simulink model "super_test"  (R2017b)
settings: Solver=FixedStepDiscrete  StartTime=0.0  StopTime=10.0  FixedStep=0.01  RelTol=1e-3
undefined symbols (not defined in the file or in its folder): BCCR_tiPwrUpCondLv_C, bin2dec, HVSR_dcHvilPwmDutyHi_C, HVSR_dcHvilPwmDutyLo_C, HVSR_dcHvilPwmDutyNrm_C, HVSR_dcHvilPwmDutyOpl_C, HVSR_dcHvilPwmDutyOptSet_C, HVSR_dcHvilPwmDutyThres_C, HVSR_fHvilPwmFrqHi_C, HVSR_fHvilPwmFrqLo_C, HVSR_tiHvilOplErr_C, HVSR_tiHvilScbErr_C, HVSR_tiHvilScgErr_C, HVSR_uKL30ThresHi_C, HVSR_uKL30ThresLo_C
libraries: simulink x41

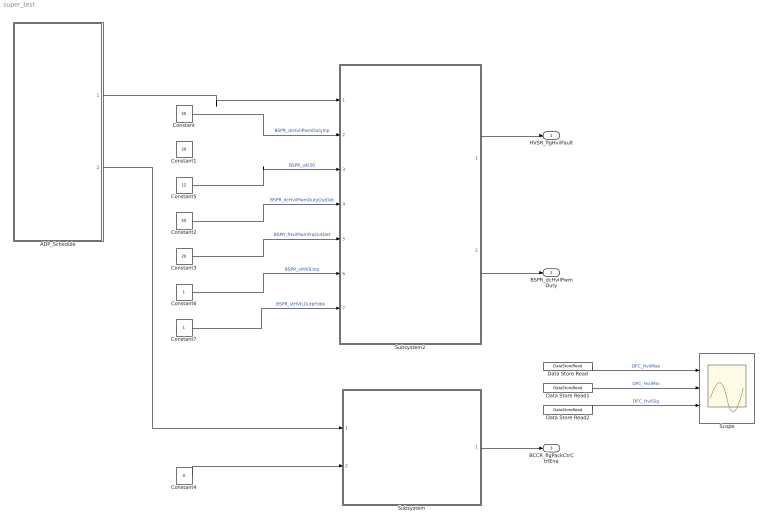
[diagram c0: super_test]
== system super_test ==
  ADP_Schedule : Stateflow chart  TreatAsAtomicUnit=on
  Constant : Constant  Value=50  OutDataTypeStr=single
  Constant1 : Constant  Value=20  OutDataTypeStr=single
  Constant2 : Constant  Value=50  OutDataTypeStr=single
  Constant3 : Constant  Value=20  OutDataTypeStr=single
  Constant4 : Constant  Value=0  OutDataTypeStr=boolean
  Constant5 : Constant  Value=12  OutDataTypeStr=single
  Constant6 : Constant  OutDataTypeStr=uint8
  Constant7 : Constant  OutDataTypeStr=uint8
  Data Store Read : DataStoreRead  DataStoreName=DFC_HvilMax
  Data Store Read1 : DataStoreRead  DataStoreName=DFC_HvilMin
  Data Store Read2 : DataStoreRead  DataStoreName=DFC_HvilSig
  Scope : Scope  NumInputPorts=3
  Subsystem : Subsystem
  Subsystem2 : Subsystem
  HVSR_flgHvilFault : Outport
  BSPR_dcHvilPwmDuty : Outport  Port=2
  BCCR_flgPackCtrCtrlEna : Outport  Port=3
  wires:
  Constant/1 -> Subsystem2/2(BSPR_dcHvilPwmDutyInp)  "BSPR_dcHvilPwmDutyInp"
  Constant1/1 -> ?  "BSPR_fHvilPwmFrq"
  Constant5/1 -> Subsystem2/3(BSPR_uKl30)  "BSPR_uKl30"
  Constant2/1 -> Subsystem2/4(BSPR_dcHvilPwmDutyOutDet)  "BSPR_dcHvilPwmDutyOutDet"
  Constant3/1 -> Subsystem2/5(BSPR_fHvilPwmFrqOutDet)  "BSPR_fHvilPwmFrqOutDet"
  Constant6/1 -> Subsystem2/6(BSPR_stHVILInp)  "BSPR_stHVILInp"
  Constant7/1 -> Subsystem2/7(BSPR_stHVILOutpFdbk)  "BSPR_stHVILOutpFdbk"
  Subsystem2/1(HVSR_flgHvilFault) -> HVSR_flgHvilFault/1
  Subsystem2/2(BSPR_dcHvilPwmDuty) -> BSPR_dcHvilPwmDuty/1
  Constant4/1 -> Subsystem/2(COMR_bKl30cLowDet)
  Subsystem/1(BCCR_flgPackCtrCtrlEna) -> BCCR_flgPackCtrCtrlEna/1
  ADP_Schedule/1(HVSR_HvilChk_step_10ms()) -> Subsystem2/1(HVSR_HvilChk_step)
  ADP_Schedule/2(BCCR_RlyCtlDiag_step_10ms()) -> Subsystem/1(BCCR_RlyCtlDiag_step)
  Data Store Read/1 -> Scope/1  "DFC_HvilMax"
  Data Store Read1/1 -> Scope/2  "DFC_HvilMin"
  Data Store Read2/1 -> Scope/3  "DFC_HvilSig"

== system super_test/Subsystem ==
  BCCR_RlyCtlDiag_step : Inport
  COMR_bKl30cLowDet : Inport  Port=2
  Subsystem1 : Subsystem
  BCCR_flgPackCtrCtrlEna : Outport
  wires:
  Subsystem1/1(BCCR_flgPackCtrCtrlEna) -> BCCR_flgPackCtrCtrlEna/1
  COMR_bKl30cLowDet/1 -> Subsystem1/1(COMR_bKl30cLowDet)
  BCCR_RlyCtlDiag_step/1 -> Subsystem1/Trigger

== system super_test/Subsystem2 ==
  HVSR_HvilChk_step : Inport
  BSPR_dcHvilPwmDutyInp : Inport  Port=2
  BSPR_uKl30 : Inport  Port=3
  BSPR_dcHvilPwmDutyOutDet : Inport  Port=4
  BSPR_fHvilPwmFrqOutDet : Inport  Port=5
  BSPR_stHVILInp : Inport  Port=6
  BSPR_stHVILOutpFdbk : Inport  Port=7
  Subsystem : Subsystem
  HVSR_flgHvilFault : Outport
  BSPR_dcHvilPwmDuty : Outport  Port=2
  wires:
  Subsystem/2(BSPR_dcHvilPwmDuty) -> BSPR_dcHvilPwmDuty/1
  Subsystem/1(HVSR_flgHvilFault) -> HVSR_flgHvilFault/1
  BSPR_stHVILOutpFdbk/1 -> Subsystem/6(BSPR_stHVILOutpFdbk)
  BSPR_stHVILInp/1 -> Subsystem/5(BSPR_stHVILInp)
  BSPR_fHvilPwmFrqOutDet/1 -> Subsystem/4(BSPR_fHvilPwmFrqOutDet)
  BSPR_dcHvilPwmDutyOutDet/1 -> Subsystem/3(BSPR_dcHvilPwmDutyOutDet)
  BSPR_uKl30/1 -> Subsystem/2(BSPR_uKl30)
  BSPR_dcHvilPwmDutyInp/1 -> Subsystem/1(BSPR_dcHvilPwmDutyInp)
  HVSR_HvilChk_step/1 -> Subsystem/Trigger

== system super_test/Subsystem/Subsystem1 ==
  COMR_bKl30cLowDet : Inport
  BCCR_RlyCtlDiag_step : TriggerPort  TriggerType=function-call  VariantControl=(inherit)
  Subsystem : Subsystem
  BCCR_flgPackCtrCtrlEna : Outport
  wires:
  COMR_bKl30cLowDet/1 -> Subsystem/1(COMR_bKl30cLowDet)
  Subsystem/1(BCCR_flgPackCtrCtrlEna) -> BCCR_flgPackCtrCtrlEna/1

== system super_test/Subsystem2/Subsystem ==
  BSPR_dcHvilPwmDutyInp : Inport
  BSPR_uKl30 : Inport  Port=2
  BSPR_dcHvilPwmDutyOutDet : Inport  Port=3
  BSPR_fHvilPwmFrqOutDet : Inport  Port=4
  BSPR_stHVILInp : Inport  Port=5
  BSPR_stHVILOutpFdbk : Inport  Port=6
  HVSR_HvilChk_step : TriggerPort  TriggerType=function-call  VariantControl=(inherit)
  HVSR_HvilChk : Subsystem
  HVSR_flgHvilFault : Outport
  BSPR_dcHvilPwmDuty : Outport  Port=2
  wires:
  BSPR_uKl30/1 -> HVSR_HvilChk/2(BSPR_uKl30)
  BSPR_dcHvilPwmDutyInp/1 -> HVSR_HvilChk/1(BSPR_dcHvilPwmDutyInp)
  BSPR_dcHvilPwmDutyOutDet/1 -> HVSR_HvilChk/3(BSPR_dcHvilPwmDutyOutDet)
  BSPR_fHvilPwmFrqOutDet/1 -> HVSR_HvilChk/4(BSPR_fHvilPwmFrqOutDet)
  BSPR_stHVILInp/1 -> HVSR_HvilChk/5(BSPR_stHVILInp)
  HVSR_HvilChk/1(HVSR_flgHvilFault) -> HVSR_flgHvilFault/1  "HVSR_flgHvilFault"
  BSPR_stHVILOutpFdbk/1 -> HVSR_HvilChk/6(BSPR_stHVILOutpFdbk)
  HVSR_HvilChk/2(BSPR_dcHvilPwmDuty) -> BSPR_dcHvilPwmDuty/1  "BSPR_dcHvilPwmDuty"

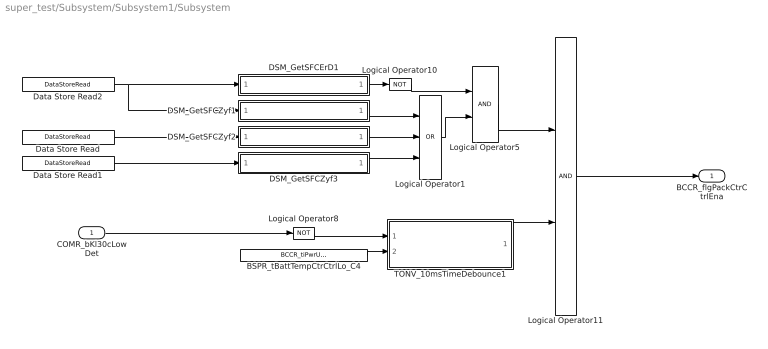
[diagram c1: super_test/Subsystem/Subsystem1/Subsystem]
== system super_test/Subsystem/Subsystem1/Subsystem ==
  COMR_bKl30cLowDet : Inport
  BSPR_tBattTempCtrCtrlLo_C4 : Constant  Value=BCCR_tiPwrUpCondLv_C
  DSM_GetSFCErD1 : Subsystem  TreatAsAtomicUnit=on  RTWFcnName=TONV_10msTimeDebounce  RTWFileName=SrvLib
  DSM_GetSFCZyf1 : Subsystem  TreatAsAtomicUnit=on  RTWFcnName=TONV_10msTimeDebounce  RTWFileName=SrvLib
  DSM_GetSFCZyf2 : Subsystem  TreatAsAtomicUnit=on  RTWFcnName=TONV_10msTimeDebounce  RTWFileName=SrvLib
  DSM_GetSFCZyf3 : Subsystem  TreatAsAtomicUnit=on  RTWFcnName=TONV_10msTimeDebounce  RTWFileName=SrvLib
  Data Store Read : DataStoreRead  DataStoreName=DFC_HvilMax
  Data Store Read1 : DataStoreRead  DataStoreName=DFC_HvilMin
  Data Store Read2 : DataStoreRead  DataStoreName=DFC_HvilSig
  Logical Operator1 : Logic  Operator=OR  Inputs=3  AllPortsSameDT=off  OutDataTypeStr=boolean
  Logical Operator10 : Logic  Operator=NOT  AllPortsSameDT=off  OutDataTypeStr=boolean
  Logical Operator11 : Logic  AllPortsSameDT=off  OutDataTypeStr=boolean
  Logical Operator5 : Logic  AllPortsSameDT=off  OutDataTypeStr=boolean
  Logical Operator8 : Logic  Operator=NOT  AllPortsSameDT=off  OutDataTypeStr=boolean
  TONV_10msTimeDebounce1 : Subsystem  TreatAsAtomicUnit=on  RTWFcnName=TONV_10msTimeDebounce  RTWFileName=SrvLib
  BCCR_flgPackCtrCtrlEna : Outport
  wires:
  Logical Operator11/1 -> BCCR_flgPackCtrCtrlEna/1
  DSM_GetSFCZyf2/1(y) -> Logical Operator1/2
  Logical Operator1/1 -> Logical Operator5/2
  TONV_10msTimeDebounce1/1(y) -> Logical Operator11/2
  Logical Operator8/1 -> TONV_10msTimeDebounce1/1(u)
  Logical Operator10/1 -> Logical Operator5/1
  DSM_GetSFCErD1/1(y) -> Logical Operator10/1
  BSPR_tBattTempCtrCtrlLo_C4/1 -> TONV_10msTimeDebounce1/2(T)
  Logical Operator5/1 -> Logical Operator11/1
  DSM_GetSFCZyf3/1(y) -> Logical Operator1/3
  COMR_bKl30cLowDet/1 -> Logical Operator8/1
  DSM_GetSFCZyf1/1(y) -> Logical Operator1/1
  Data Store Read1/1 -> DSM_GetSFCZyf3/1(DFC)
  Data Store Read2/1 -> DSM_GetSFCZyf1/1(DFC), DSM_GetSFCErD1/1(DFC)
  Data Store Read/1 -> DSM_GetSFCZyf2/1(DFC)

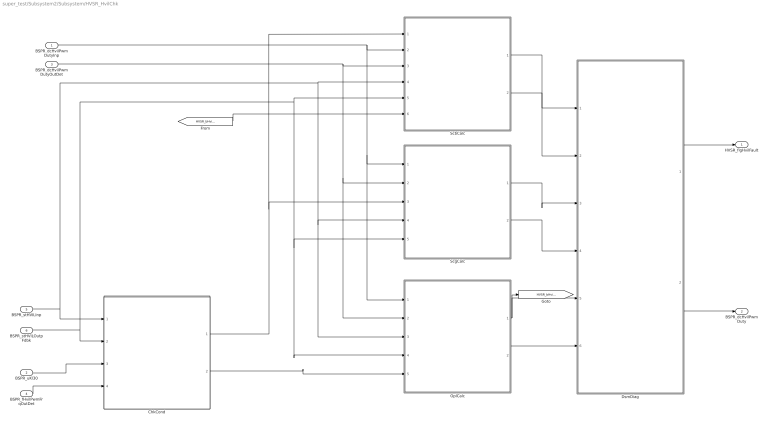
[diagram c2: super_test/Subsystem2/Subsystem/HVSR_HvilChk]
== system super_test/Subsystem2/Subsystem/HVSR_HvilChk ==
  BSPR_dcHvilPwmDutyInp : Inport
  BSPR_uKl30 : Inport  Port=2
  BSPR_dcHvilPwmDutyOutDet : Inport  Port=3
  BSPR_fHvilPwmFrqOutDet : Inport  Port=4
  BSPR_stHVILInp : Inport  Port=5
  BSPR_stHVILOutpFdbk : Inport  Port=6
  ChkCond : Subsystem
  DsmDiag : Subsystem
  OplCalc : Subsystem
  ScbCalc : Subsystem
  ScgCalc : Subsystem
  HVSR_flgHvilFault : Outport
  BSPR_dcHvilPwmDuty : Outport  Port=2
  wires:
  BSPR_uKl30/1 -> ChkCond/3(BSPR_uKl30)
  BSPR_dcHvilPwmDutyInp/1 -> ScgCalc/1(BSPR_dcHvilPwmDutyInp), OplCalc/1(BSPR_dcHvilPwmDutyInp), ScbCalc/2(BSPR_dcHvilPwmDutyInp)
  ScgCalc/1(HVSR_bHvilScgErrDet) -> DsmDiag/3(HVSR_bHvilScgErrDet)
  ScgCalc/2(HVSR_bHvilScgErrHeal) -> DsmDiag/4(HVSR_bHvilScgErrHeal)
  ChkCond/1(BSPR_bKl30HvilDiagCond) -> ScbCalc/1(BSPR_bKl30HvilDiagCond), ScgCalc/3(BSPR_bKl30HvilDiagCond)
  ScbCalc/1(HVSR_bHvilScbErrDet) -> DsmDiag/1(HVSR_bHvilScbErrDet)
  ScbCalc/2(HVSR_bHvilScbErrHeal) -> DsmDiag/2(HVSR_bHvilScbErrHeal)
  DsmDiag/1(HVSR_flgHvilFault) -> HVSR_flgHvilFault/1
  OplCalc/2(HVSR_bHvilOplErrHeal) -> DsmDiag/6(HVSR_bHvilOplErrHeal)
  OplCalc/1(HVSR_bHvilOplErrDet) -> [HVSR_bHvilOplErrDet], DsmDiag/5(HVSR_bHvilOplErrDet)
  ChkCond/2(BSPR_bHvilDiagCond) -> OplCalc/5(BSPR_bHvilDiagCond)
  BSPR_dcHvilPwmDutyOutDet/1 -> ScgCalc/2(BSPR_dcHvilPwmDutyOutDet), OplCalc/2(BSPR_dcHvilPwmDutyOutDet), ScbCalc/3(BSPR_dcHvilPwmDutyOutDet)
  BSPR_fHvilPwmFrqOutDet/1 -> ChkCond/4(BSPR_fHvilPwmFrqOutDet)
  BSPR_stHVILInp/1 -> ChkCond/1(BSPR_stHVILInp), ScgCalc/4(BSPR_stHVILInp), OplCalc/3(BSPR_stHVILInp), ScbCalc/4(BSPR_stHVILInp)
  BSPR_stHVILOutpFdbk/1 -> ChkCond/2(BSPR_stHVILOutpFdbk), ScgCalc/5(BSPR_stHVILOutpFdbk), OplCalc/4(BSPR_stHVILOutpFdbk), ScbCalc/5(BSPR_stHVILOutpFdbk)
  DsmDiag/2(BSPR_dcHvilPwmDuty) -> BSPR_dcHvilPwmDuty/1
  [HVSR_bHvilOplErrDet] -> ScbCalc/6(HVSR_bHvilOplErrDet)

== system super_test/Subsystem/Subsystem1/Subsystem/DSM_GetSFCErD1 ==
  DFC : Inport  OutDataTypeStr=uint8
  DFC_IsoChkLv1_1 : simulink/Logic and Bit Operations/Bitwise Operator  logicop=AND  UseBitMask=on  BitMask=bin2dec('00010000')  BitMaskRealWorld=Stored Integer
  DFC_IsoChkLv1_1_compare : simulink/Logic and Bit Operations/Compare To Constant  relop===  const=16  OutDataTypeStr=boolean
  y : Outport
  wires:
  DFC_IsoChkLv1_1_compare/1 -> y/1
  DFC/1 -> DFC_IsoChkLv1_1/1
  DFC_IsoChkLv1_1/1 -> DFC_IsoChkLv1_1_compare/1

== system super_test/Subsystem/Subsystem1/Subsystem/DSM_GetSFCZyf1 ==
  DFC : Inport  OutDataTypeStr=uint8
  DFC_IsoChkLv1_1 : simulink/Logic and Bit Operations/Bitwise Operator  logicop=AND  UseBitMask=on  BitMask=bin2dec('00001000')  BitMaskRealWorld=Stored Integer
  DFC_IsoChkLv1_1_compare1 : simulink/Logic and Bit Operations/Compare To Constant  relop===  const=8  OutDataTypeStr=boolean
  y : Outport
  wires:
  DFC_IsoChkLv1_1_compare1/1 -> y/1
  DFC/1 -> DFC_IsoChkLv1_1/1
  DFC_IsoChkLv1_1/1 -> DFC_IsoChkLv1_1_compare1/1

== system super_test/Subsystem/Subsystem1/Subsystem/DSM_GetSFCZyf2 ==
  DFC : Inport  OutDataTypeStr=uint8
  DFC_IsoChkLv1_1 : simulink/Logic and Bit Operations/Bitwise Operator  logicop=AND  UseBitMask=on  BitMask=bin2dec('00001000')  BitMaskRealWorld=Stored Integer
  DFC_IsoChkLv1_1_compare1 : simulink/Logic and Bit Operations/Compare To Constant  relop===  const=8  OutDataTypeStr=boolean
  y : Outport
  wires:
  DFC_IsoChkLv1_1/1 -> DFC_IsoChkLv1_1_compare1/1
  DFC/1 -> DFC_IsoChkLv1_1/1
  DFC_IsoChkLv1_1_compare1/1 -> y/1

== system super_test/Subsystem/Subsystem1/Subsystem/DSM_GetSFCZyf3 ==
  DFC : Inport  OutDataTypeStr=uint8
  DFC_IsoChkLv1_1 : simulink/Logic and Bit Operations/Bitwise Operator  logicop=AND  UseBitMask=on  BitMask=bin2dec('00001000')  BitMaskRealWorld=Stored Integer
  DFC_IsoChkLv1_1_compare1 : simulink/Logic and Bit Operations/Compare To Constant  relop===  const=8  OutDataTypeStr=boolean
  y : Outport
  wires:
  DFC_IsoChkLv1_1_compare1/1 -> y/1
  DFC/1 -> DFC_IsoChkLv1_1/1
  DFC_IsoChkLv1_1/1 -> DFC_IsoChkLv1_1_compare1/1

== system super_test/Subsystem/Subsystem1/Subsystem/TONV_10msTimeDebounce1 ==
  note: Turn On Delay Time Deboune
  u : Inport
  T : Inport  Port=2
  Add : Sum
  Constant1 : Constant  Value=0  OutDataTypeStr=single
  Constant2 : Constant  OutDataTypeStr=uint8
  Constant3 : Constant  Value=0  OutDataTypeStr=uint8
  Constant4 : Constant  Value=0.01  OutDataTypeStr=single
  Delay : Delay  DelayLength=1  InitialCondition=0
  MinMax : MinMax  Inputs=2
  Product : Product  OutMin=[0]  OutMax=[65535]  OutDataTypeStr=single
  Relational Operator : RelationalOperator  Operator=>  OutDataTypeStr=boolean  RndMeth=Simplest
  Switch : Switch  Criteria=u2 ~= 0
  Switch1 : Switch  Criteria=u2 ~= 0
  y : Outport
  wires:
  MinMax/1 -> Add/2
  T/1 -> Relational Operator/2, MinMax/1
  Relational Operator/1 -> y/1
  Delay/1 -> MinMax/2
  Switch/1 -> Add/1
  Product/1 -> Delay/1, Relational Operator/1
  Add/1 -> Product/2
  Constant1/1 -> Switch/3
  Constant4/1 -> Switch/1
  u/1 -> Switch/2, Switch1/2
  Constant2/1 -> Switch1/1
  Constant3/1 -> Switch1/3
  Switch1/1 -> Product/1

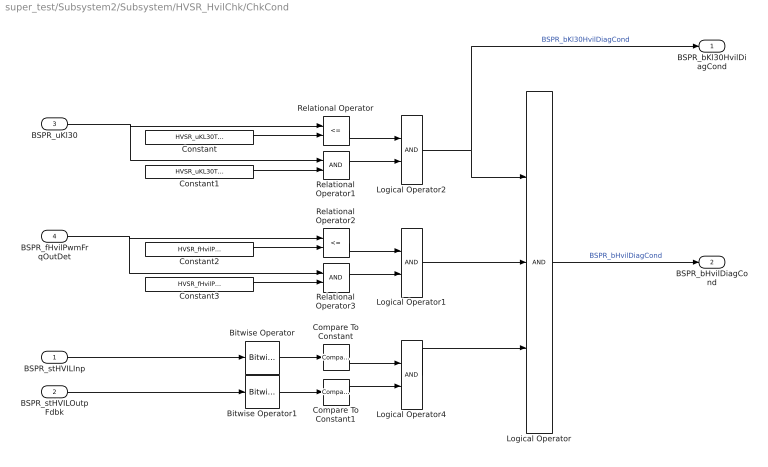
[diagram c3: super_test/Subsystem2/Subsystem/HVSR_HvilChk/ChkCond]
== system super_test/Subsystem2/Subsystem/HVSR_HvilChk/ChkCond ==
  BSPR_stHVILInp : Inport
  BSPR_stHVILOutpFdbk : Inport  Port=2
  BSPR_uKl30 : Inport  Port=3
  BSPR_fHvilPwmFrqOutDet : Inport  Port=4
  Bitwise Operator : simulink/Logic and Bit Operations/Bitwise Operator  logicop=AND  UseBitMask=on  BitMask=bin2dec('00010000')  BitMaskRealWorld=Stored Integer
  Bitwise Operator1 : simulink/Logic and Bit Operations/Bitwise Operator  logicop=AND  UseBitMask=on  BitMask=bin2dec('00010000')  BitMaskRealWorld=Stored Integer
  Compare To Constant : simulink/Logic and Bit Operations/Compare To Constant  relop===  const=0  OutDataTypeStr=boolean
  Compare To Constant1 : simulink/Logic and Bit Operations/Compare To Constant  relop===  const=0  OutDataTypeStr=boolean
  Constant : Constant  Value=HVSR_uKL30ThresHi_C
  Constant1 : Constant  Value=HVSR_uKL30ThresLo_C
  Constant2 : Constant  Value=HVSR_fHvilPwmFrqHi_C
  Constant3 : Constant  Value=HVSR_fHvilPwmFrqLo_C
  Logical Operator : Logic  Inputs=3  AllPortsSameDT=off  OutDataTypeStr=boolean
  Logical Operator1 : Logic  AllPortsSameDT=off  OutDataTypeStr=boolean
  Logical Operator2 : Logic  AllPortsSameDT=off  OutDataTypeStr=boolean
  Logical Operator4 : Logic  AllPortsSameDT=off  OutDataTypeStr=boolean
  Relational Operator : RelationalOperator  Operator=<=  OutDataTypeStr=boolean  RndMeth=Simplest
  Relational Operator1 : RelationalOperator  OutDataTypeStr=boolean  RndMeth=Simplest
  Relational Operator2 : RelationalOperator  Operator=<=  OutDataTypeStr=boolean  RndMeth=Simplest
  Relational Operator3 : RelationalOperator  OutDataTypeStr=boolean  RndMeth=Simplest
  BSPR_bKl30HvilDiagCond : Outport
  BSPR_bHvilDiagCond : Outport  Port=2
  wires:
  BSPR_uKl30/1 -> Relational Operator/1, Relational Operator1/1
  Logical Operator/1 -> BSPR_bHvilDiagCond/1  "BSPR_bHvilDiagCond"
  Constant/1 -> Relational Operator/2
  Constant1/1 -> Relational Operator1/2
  BSPR_fHvilPwmFrqOutDet/1 -> Relational Operator2/1, Relational Operator3/1
  Relational Operator/1 -> Logical Operator2/1
  Relational Operator1/1 -> Logical Operator2/2
  Logical Operator2/1 -> BSPR_bKl30HvilDiagCond/1, Logical Operator/1  "BSPR_bKl30HvilDiagCond"
  Constant2/1 -> Relational Operator2/2
  Constant3/1 -> Relational Operator3/2
  Relational Operator2/1 -> Logical Operator1/1
  Relational Operator3/1 -> Logical Operator1/2
  Logical Operator1/1 -> Logical Operator/2
  BSPR_stHVILInp/1 -> Bitwise Operator/1
  BSPR_stHVILOutpFdbk/1 -> Bitwise Operator1/1
  Bitwise Operator/1 -> Compare To Constant/1
  Bitwise Operator1/1 -> Compare To Constant1/1
  Compare To Constant/1 -> Logical Operator4/1
  Compare To Constant1/1 -> Logical Operator4/2
  Logical Operator4/1 -> Logical Operator/3

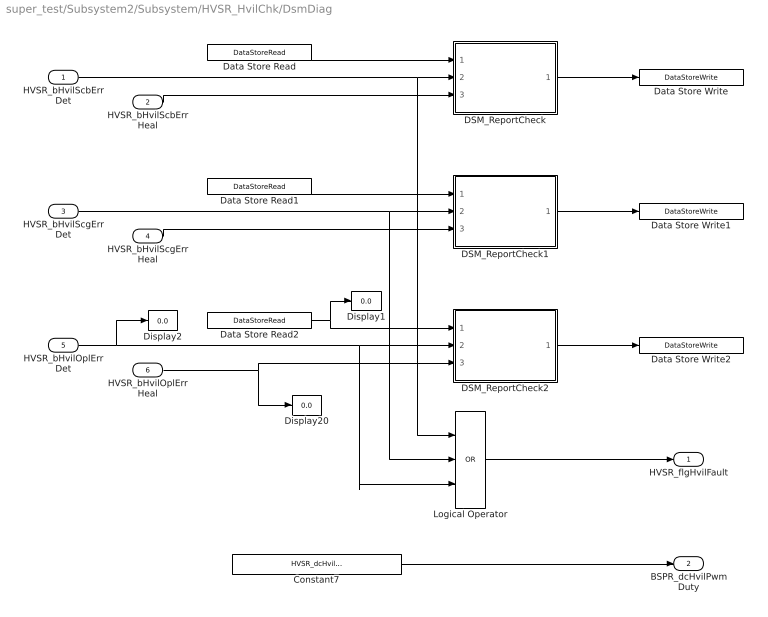
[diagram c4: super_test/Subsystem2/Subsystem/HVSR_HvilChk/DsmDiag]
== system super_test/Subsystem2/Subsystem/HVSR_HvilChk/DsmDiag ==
  HVSR_bHvilScbErrDet : Inport
  HVSR_bHvilScbErrHeal : Inport  Port=2
  HVSR_bHvilScgErrDet : Inport  Port=3
  HVSR_bHvilScgErrHeal : Inport  Port=4
  HVSR_bHvilOplErrDet : Inport  Port=5
  HVSR_bHvilOplErrHeal : Inport  Port=6
  Constant7 : Constant  Value=HVSR_dcHvilPwmDutyOptSet_C
  DSM_ReportCheck : Subsystem  TreatAsAtomicUnit=on  RTWFcnName=DSM_ReportCheck  RTWFileName=SrvLib
  DSM_ReportCheck1 : Subsystem  TreatAsAtomicUnit=on  RTWFcnName=DSM_ReportCheck  RTWFileName=SrvLib
  DSM_ReportCheck2 : Subsystem  TreatAsAtomicUnit=on  RTWFcnName=DSM_ReportCheck  RTWFileName=SrvLib
  Data Store Read : DataStoreRead  DataStoreName=DFC_HvilMax
  Data Store Read1 : DataStoreRead  DataStoreName=DFC_HvilMin
  Data Store Read2 : DataStoreRead  DataStoreName=DFC_HvilSig
  Data Store Write : DataStoreWrite  DataStoreName=DFC_HvilMax
  Data Store Write1 : DataStoreWrite  DataStoreName=DFC_HvilMin
  Data Store Write2 : DataStoreWrite  DataStoreName=DFC_HvilSig
  Display1 : Display
  Display2 : Display
  Display20 : Display
  Logical Operator : Logic  Operator=OR  Inputs=3  AllPortsSameDT=off  OutDataTypeStr=boolean
  HVSR_flgHvilFault : Outport
  BSPR_dcHvilPwmDuty : Outport  Port=2
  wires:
  Data Store Read1/1 -> DSM_ReportCheck1/1(Dfc_id_nv)
  DSM_ReportCheck2/1(Dfc_id) -> Data Store Write2/1
  Data Store Read/1 -> DSM_ReportCheck/1(Dfc_id_nv)
  Data Store Read2/1 -> Display1/1, DSM_ReportCheck2/1(Dfc_id_nv)
  DSM_ReportCheck1/1(Dfc_id) -> Data Store Write1/1
  DSM_ReportCheck/1(Dfc_id) -> Data Store Write/1
  HVSR_bHvilScbErrHeal/1 -> DSM_ReportCheck/3(Heal)
  HVSR_bHvilScbErrDet/1 -> DSM_ReportCheck/2(Err), Logical Operator/1
  HVSR_bHvilScgErrHeal/1 -> DSM_ReportCheck1/3(Heal)
  HVSR_bHvilScgErrDet/1 -> DSM_ReportCheck1/2(Err), Logical Operator/2
  HVSR_bHvilOplErrHeal/1 -> Display20/1, DSM_ReportCheck2/3(Heal)
  HVSR_bHvilOplErrDet/1 -> Display2/1, DSM_ReportCheck2/2(Err), Logical Operator/3
  Logical Operator/1 -> HVSR_flgHvilFault/1
  Constant7/1 -> BSPR_dcHvilPwmDuty/1

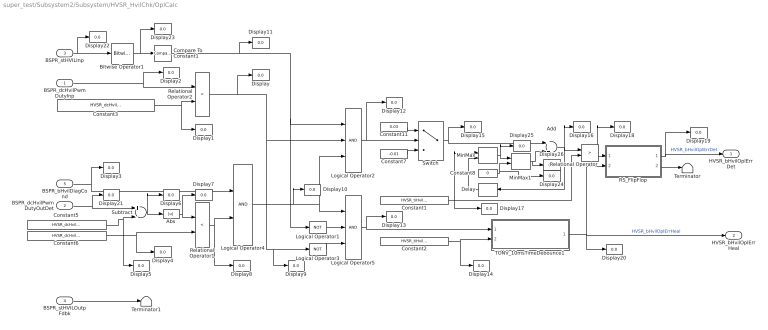
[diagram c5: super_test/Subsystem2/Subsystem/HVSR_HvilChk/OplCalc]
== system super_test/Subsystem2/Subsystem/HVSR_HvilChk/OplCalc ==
  BSPR_dcHvilPwmDutyInp : Inport
  BSPR_dcHvilPwmDutyOutDet : Inport  Port=2
  BSPR_stHVILInp : Inport  Port=3
  BSPR_stHVILOutpFdbk : Inport  Port=4
  BSPR_bHvilDiagCond : Inport  Port=5
  Abs : Abs
  Add : Sum
  Bitwise Operator1 : simulink/Logic and Bit Operations/Bitwise Operator  logicop=AND  UseBitMask=on  BitMask=bin2dec('00001000')  BitMaskRealWorld=Stored Integer
  Compare To Constant1 : simulink/Logic and Bit Operations/Compare To Constant  relop===  const=8  OutDataTypeStr=boolean
  Constant1 : Constant  Value=HVSR_tiHvilOplErr_C
  Constant11 : Constant  Value=0.03  OutDataTypeStr=single
  Constant2 : Constant  Value=HVSR_tiHvilOplErr_C
  Constant3 : Constant  Value=HVSR_dcHvilPwmDutyOpl_C
  Constant5 : Constant  Value=HVSR_dcHvilPwmDutyNrm_C
  Constant6 : Constant  Value=HVSR_dcHvilPwmDutyThres_C
  Constant7 : Constant  Value=-0.01  OutDataTypeStr=single
  Constant8 : Constant  Value=0  OutDataTypeStr=single
  Delay : Delay  DelayLength=1  InitialCondition=0
  Display{,1..26} (27 alike) : Display
  Logical Operator1 : Logic  Operator=NOT  AllPortsSameDT=off  OutDataTypeStr=boolean
  Logical Operator2 : Logic  Inputs=3  AllPortsSameDT=off  OutDataTypeStr=boolean
  Logical Operator3 : Logic  Operator=NOT  AllPortsSameDT=off  OutDataTypeStr=boolean
  Logical Operator4 : Logic  AllPortsSameDT=off  OutDataTypeStr=boolean
  Logical Operator5 : Logic  Inputs=3  AllPortsSameDT=off  OutDataTypeStr=boolean
  MinMax : MinMax  Inputs=2
  MinMax1 : MinMax  Function=max  Inputs=2
  RS_FlipFlop : Subsystem
  Relational Operator : RelationalOperator  Operator=>  OutDataTypeStr=boolean  RndMeth=Simplest
  Relational Operator1 : RelationalOperator  Operator=<  OutDataTypeStr=boolean  RndMeth=Simplest
  Relational Operator2 : RelationalOperator  Operator=<  OutDataTypeStr=boolean  RndMeth=Simplest
  Subtract : Sum  Inputs=+-
  Switch : Switch  Criteria=u2 ~= 0
  TONV_10msTimeDebounce1 : Subsystem  TreatAsAtomicUnit=on  RTWFcnName=TONV_10msTimeDebounce  RTWFileName=SrvLib
  Terminator : Terminator
  Terminator1 : Terminator
  HVSR_bHvilOplErrDet : Outport
  HVSR_bHvilOplErrHeal : Outport  Port=2
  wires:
  BSPR_bHvilDiagCond/1 -> Display3/1, Logical Operator4/1
  Logical Operator5/1 -> Display13/1, TONV_10msTimeDebounce1/1(u)
  Constant2/1 -> Display14/1, TONV_10msTimeDebounce1/2(T)
  Subtract/1 -> Display6/1, Abs/1
  Constant5/1 -> Display5/1, Subtract/2
  Abs/1 -> Display7/1, Relational Operator1/1
  Constant6/1 -> Display4/1, Relational Operator1/2
  Relational Operator1/1 -> Display8/1, Logical Operator4/2
  Relational Operator2/1 -> Display/1, Logical Operator2/2, Display9/1, Logical Operator3/1
  MinMax1/1 -> Display26/1, Add/2
  Constant1/1 -> Relational Operator/2, Display17/1, MinMax/1
  Delay/1 -> MinMax/2
  Switch/1 -> Display15/1, Add/1
  Add/1 -> Display16/1, Delay/1, Relational Operator/1
  Constant7/1 -> Switch/3
  Constant11/1 -> Switch/1
  MinMax/1 -> Display25/1, MinMax1/1
  Constant8/1 -> Display24/1, MinMax1/2
  Logical Operator2/1 -> Display12/1, Switch/2
  Relational Operator/1 -> Display18/1, RS_FlipFlop/1(S)
  Logical Operator3/1 -> Logical Operator5/3
  Logical Operator4/1 -> Logical Operator5/1, Logical Operator2/3, Display10/1
  TONV_10msTimeDebounce1/1(y) -> Display20/1, HVSR_bHvilOplErrHeal/1, RS_FlipFlop/2(R)  "HVSR_bHvilOplErrHeal"
  RS_FlipFlop/2(!Q) -> Terminator/1
  RS_FlipFlop/1(Q) -> Display19/1, HVSR_bHvilOplErrDet/1  "HVSR_bHvilOplErrDet"
  BSPR_dcHvilPwmDutyOutDet/1 -> Display21/1, Subtract/1
  BSPR_dcHvilPwmDutyInp/1 -> Display2/1, Relational Operator2/1
  Constant3/1 -> Display1/1, Relational Operator2/2
  Bitwise Operator1/1 -> Display23/1, Compare To Constant1/1
  BSPR_stHVILInp/1 -> Display22/1, Bitwise Operator1/1
  BSPR_stHVILOutpFdbk/1 -> Terminator1/1
  Compare To Constant1/1 -> Display11/1, Logical Operator2/1, Logical Operator1/1
  Logical Operator1/1 -> Logical Operator5/2

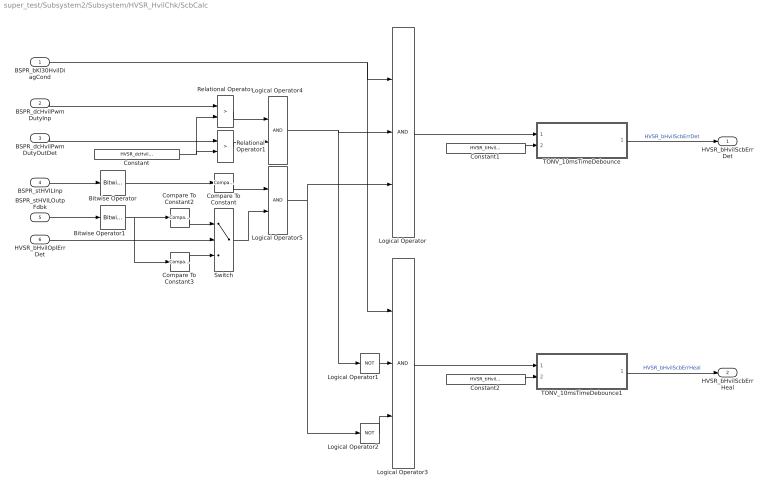
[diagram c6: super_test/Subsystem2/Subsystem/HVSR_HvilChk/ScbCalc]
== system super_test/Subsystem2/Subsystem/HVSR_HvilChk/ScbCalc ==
  BSPR_bKl30HvilDiagCond : Inport
  BSPR_dcHvilPwmDutyInp : Inport  Port=2
  BSPR_dcHvilPwmDutyOutDet : Inport  Port=3
  BSPR_stHVILInp : Inport  Port=4
  BSPR_stHVILOutpFdbk : Inport  Port=5
  HVSR_bHvilOplErrDet : Inport  Port=6
  Bitwise Operator : simulink/Logic and Bit Operations/Bitwise Operator  logicop=AND  UseBitMask=on  BitMask=bin2dec('00001001')  BitMaskRealWorld=Stored Integer
  Bitwise Operator1 : simulink/Logic and Bit Operations/Bitwise Operator  logicop=AND  UseBitMask=on  BitMask=bin2dec('00001001')  BitMaskRealWorld=Stored Integer
  Compare To Constant : simulink/Logic and Bit Operations/Compare To Constant  relop===  const=9  OutDataTypeStr=boolean
  Compare To Constant2 : simulink/Logic and Bit Operations/Compare To Constant  relop===  const=8  OutDataTypeStr=boolean
  Compare To Constant3 : simulink/Logic and Bit Operations/Compare To Constant  relop===  const=9  OutDataTypeStr=boolean
  Constant : Constant  Value=HVSR_dcHvilPwmDutyHi_C
  Constant1 : Constant  Value=HVSR_tiHvilScbErr_C
  Constant2 : Constant  Value=HVSR_tiHvilScbErr_C
  Logical Operator : Logic  Inputs=3  AllPortsSameDT=off  OutDataTypeStr=boolean
  Logical Operator1 : Logic  Operator=NOT  AllPortsSameDT=off  OutDataTypeStr=boolean
  Logical Operator2 : Logic  Operator=NOT  AllPortsSameDT=off  OutDataTypeStr=boolean
  Logical Operator3 : Logic  Inputs=3  AllPortsSameDT=off  OutDataTypeStr=boolean
  Logical Operator4 : Logic  AllPortsSameDT=off  OutDataTypeStr=boolean
  Logical Operator5 : Logic  AllPortsSameDT=off  OutDataTypeStr=boolean
  Relational Operator : RelationalOperator  Operator=>  OutDataTypeStr=boolean  RndMeth=Simplest
  Relational Operator1 : RelationalOperator  Operator=>  OutDataTypeStr=boolean  RndMeth=Simplest
  Switch : Switch  Criteria=u2 ~= 0
  TONV_10msTimeDebounce : Subsystem  TreatAsAtomicUnit=on  RTWFcnName=TONV_10msTimeDebounce  RTWFileName=SrvLib
  TONV_10msTimeDebounce1 : Subsystem  TreatAsAtomicUnit=on  RTWFcnName=TONV_10msTimeDebounce  RTWFileName=SrvLib
  HVSR_bHvilScbErrDet : Outport
  HVSR_bHvilScbErrHeal : Outport  Port=2
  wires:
  Logical Operator2/1 -> Logical Operator3/3
  TONV_10msTimeDebounce1/1(y) -> HVSR_bHvilScbErrHeal/1  "HVSR_bHvilScbErrHeal"
  Logical Operator3/1 -> TONV_10msTimeDebounce1/1(u)
  Constant2/1 -> TONV_10msTimeDebounce1/2(T)
  BSPR_bKl30HvilDiagCond/1 -> Logical Operator/1, Logical Operator3/1
  Constant1/1 -> TONV_10msTimeDebounce/2(T)
  Logical Operator/1 -> TONV_10msTimeDebounce/1(u)
  Constant/1 -> Relational Operator/2, Relational Operator1/2
  BSPR_dcHvilPwmDutyInp/1 -> Relational Operator/1
  TONV_10msTimeDebounce/1(y) -> HVSR_bHvilScbErrDet/1  "HVSR_bHvilScbErrDet"
  BSPR_dcHvilPwmDutyOutDet/1 -> Relational Operator1/1
  Logical Operator1/1 -> Logical Operator3/2
  Bitwise Operator/1 -> Compare To Constant/1
  BSPR_stHVILInp/1 -> Bitwise Operator/1
  BSPR_stHVILOutpFdbk/1 -> Bitwise Operator1/1
  Relational Operator1/1 -> Logical Operator4/2
  Relational Operator/1 -> Logical Operator4/1
  Logical Operator4/1 -> Logical Operator/2, Logical Operator1/1
  Compare To Constant/1 -> Logical Operator5/1
  Logical Operator5/1 -> Logical Operator/3, Logical Operator2/1
  HVSR_bHvilOplErrDet/1 -> Switch/2
  Bitwise Operator1/1 -> Compare To Constant2/1, Compare To Constant3/1
  Compare To Constant2/1 -> Switch/1
  Compare To Constant3/1 -> Switch/3
  Switch/1 -> Logical Operator5/2

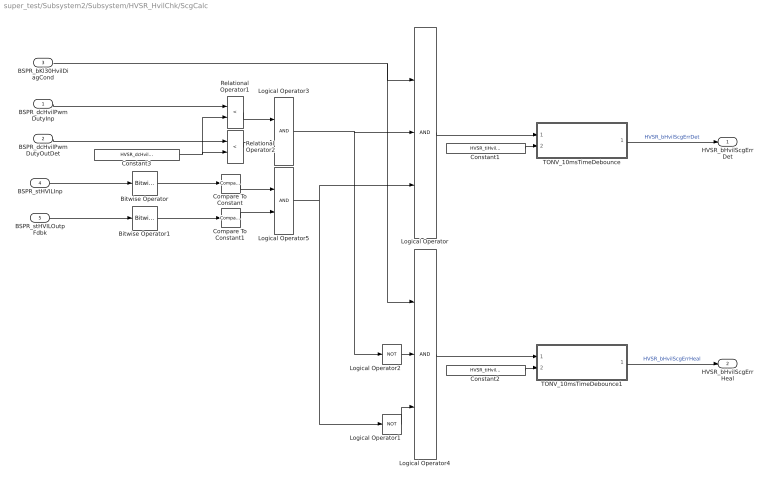
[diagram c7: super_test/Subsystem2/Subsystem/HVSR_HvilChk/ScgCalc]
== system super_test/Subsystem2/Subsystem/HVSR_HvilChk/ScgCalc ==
  BSPR_dcHvilPwmDutyInp : Inport
  BSPR_dcHvilPwmDutyOutDet : Inport  Port=2
  BSPR_bKl30HvilDiagCond : Inport  Port=3
  BSPR_stHVILInp : Inport  Port=4
  BSPR_stHVILOutpFdbk : Inport  Port=5
  Bitwise Operator : simulink/Logic and Bit Operations/Bitwise Operator  logicop=AND  UseBitMask=on  BitMask=bin2dec('00001001')  BitMaskRealWorld=Stored Integer
  Bitwise Operator1 : simulink/Logic and Bit Operations/Bitwise Operator  logicop=AND  UseBitMask=on  BitMask=bin2dec('00001001')  BitMaskRealWorld=Stored Integer
  Compare To Constant : simulink/Logic and Bit Operations/Compare To Constant  relop===  const=8  OutDataTypeStr=boolean
  Compare To Constant1 : simulink/Logic and Bit Operations/Compare To Constant  relop===  const=8  OutDataTypeStr=boolean
  Constant1 : Constant  Value=HVSR_tiHvilScgErr_C
  Constant2 : Constant  Value=HVSR_tiHvilScgErr_C
  Constant3 : Constant  Value=HVSR_dcHvilPwmDutyLo_C
  Logical Operator : Logic  Inputs=3  AllPortsSameDT=off  OutDataTypeStr=boolean
  Logical Operator1 : Logic  Operator=NOT  AllPortsSameDT=off  OutDataTypeStr=boolean
  Logical Operator2 : Logic  Operator=NOT  AllPortsSameDT=off  OutDataTypeStr=boolean
  Logical Operator3 : Logic  AllPortsSameDT=off  OutDataTypeStr=boolean
  Logical Operator4 : Logic  Inputs=3  AllPortsSameDT=off  OutDataTypeStr=boolean
  Logical Operator5 : Logic  AllPortsSameDT=off  OutDataTypeStr=boolean
  Relational Operator1 : RelationalOperator  Operator=<  OutDataTypeStr=boolean  RndMeth=Simplest
  Relational Operator2 : RelationalOperator  Operator=<  OutDataTypeStr=boolean  RndMeth=Simplest
  TONV_10msTimeDebounce : Subsystem  TreatAsAtomicUnit=on  RTWFcnName=TONV_10msTimeDebounce  RTWFileName=SrvLib
  TONV_10msTimeDebounce1 : Subsystem  TreatAsAtomicUnit=on  RTWFcnName=TONV_10msTimeDebounce  RTWFileName=SrvLib
  HVSR_bHvilScgErrDet : Outport
  HVSR_bHvilScgErrHeal : Outport  Port=2
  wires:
  TONV_10msTimeDebounce/1(y) -> HVSR_bHvilScgErrDet/1  "HVSR_bHvilScgErrDet"
  Constant1/1 -> TONV_10msTimeDebounce/2(T)
  Constant2/1 -> TONV_10msTimeDebounce1/2(T)
  TONV_10msTimeDebounce1/1(y) -> HVSR_bHvilScgErrHeal/1  "HVSR_bHvilScgErrHeal"
  Logical Operator4/1 -> TONV_10msTimeDebounce1/1(u)
  Logical Operator/1 -> TONV_10msTimeDebounce/1(u)
  Constant3/1 -> Relational Operator1/2, Relational Operator2/2
  BSPR_bKl30HvilDiagCond/1 -> Logical Operator4/1, Logical Operator/1
  BSPR_dcHvilPwmDutyInp/1 -> Relational Operator1/1
  Logical Operator2/1 -> Logical Operator4/2
  BSPR_dcHvilPwmDutyOutDet/1 -> Relational Operator2/1
  Logical Operator1/1 -> Logical Operator4/3
  Bitwise Operator/1 -> Compare To Constant/1
  Bitwise Operator1/1 -> Compare To Constant1/1
  Compare To Constant/1 -> Logical Operator5/1
  Compare To Constant1/1 -> Logical Operator5/2
  BSPR_stHVILInp/1 -> Bitwise Operator/1
  BSPR_stHVILOutpFdbk/1 -> Bitwise Operator1/1
  Relational Operator1/1 -> Logical Operator3/1
  Relational Operator2/1 -> Logical Operator3/2
  Logical Operator3/1 -> Logical Operator2/1, Logical Operator/2
  Logical Operator5/1 -> Logical Operator1/1, Logical Operator/3

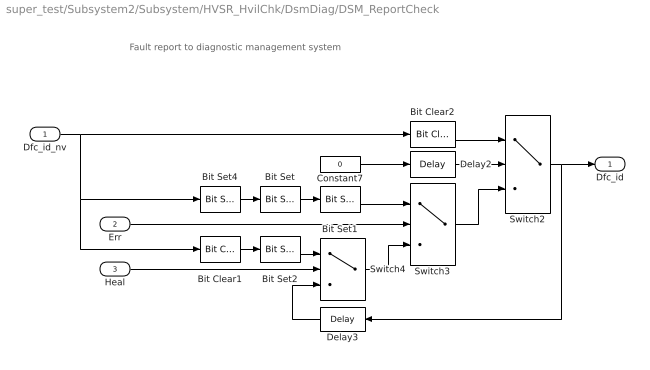
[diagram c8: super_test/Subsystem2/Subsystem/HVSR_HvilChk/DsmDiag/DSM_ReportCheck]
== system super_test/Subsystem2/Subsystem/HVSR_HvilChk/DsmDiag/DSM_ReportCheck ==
  note: Fault report to diagnostic management system
  Dfc_id_nv : Inport  OutDataTypeStr=uint8
  Err : Inport  Port=2
  Heal : Inport  Port=3
  Bit Clear1 : simulink/Logic and Bit Operations/Bit Clear  iBit=4
  Bit Clear2 : simulink/Logic and Bit Operations/Bit Clear  iBit=3
  Bit Set : simulink/Logic and Bit Operations/Bit Set  iBit=4
  Bit Set1 : simulink/Logic and Bit Operations/Bit Set  iBit=3
  Bit Set2 : simulink/Logic and Bit Operations/Bit Set  iBit=3
  Bit Set4 : simulink/Logic and Bit Operations/Bit Set  iBit=7
  Constant7 : Constant  Value=0  OutDataTypeStr=boolean
  Delay2 : Delay  DelayLength=1  InitialCondition=1
  Delay3 : Delay  DelayLength=1  InitialCondition=0
  Switch2 : Switch  Criteria=u2 ~= 0
  Switch3 : Switch  Criteria=u2 ~= 0
  Switch4 : Switch  Criteria=u2 ~= 0
  Dfc_id : Outport  OutDataTypeStr=uint8
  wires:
  Dfc_id_nv/1 -> Bit Clear2/1, Bit Set4/1, Bit Clear1/1
  Bit Set4/1 -> Bit Set/1
  Constant7/1 -> Delay2/1
  Delay2/1 -> Switch2/2
  Switch3/1 -> Switch2/3
  Bit Clear2/1 -> Switch2/1
  Switch2/1 -> Delay3/1, Dfc_id/1
  Bit Set1/1 -> Switch3/1
  Bit Set/1 -> Bit Set1/1
  Switch4/1 -> Switch3/3
  Err/1 -> Switch3/2
  Bit Set2/1 -> Switch4/1
  Bit Clear1/1 -> Bit Set2/1
  Delay3/1 -> Switch4/3
  Heal/1 -> Switch4/2

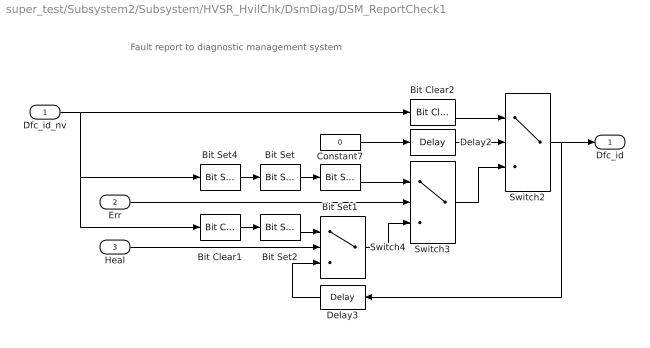
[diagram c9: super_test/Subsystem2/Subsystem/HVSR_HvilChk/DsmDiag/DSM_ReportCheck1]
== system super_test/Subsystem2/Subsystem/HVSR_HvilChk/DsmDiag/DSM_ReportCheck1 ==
  note: Fault report to diagnostic management system
  Dfc_id_nv : Inport  OutDataTypeStr=uint8
  Err : Inport  Port=2
  Heal : Inport  Port=3
  Bit Clear1 : simulink/Logic and Bit Operations/Bit Clear  iBit=4
  Bit Clear2 : simulink/Logic and Bit Operations/Bit Clear  iBit=3
  Bit Set : simulink/Logic and Bit Operations/Bit Set  iBit=4
  Bit Set1 : simulink/Logic and Bit Operations/Bit Set  iBit=3
  Bit Set2 : simulink/Logic and Bit Operations/Bit Set  iBit=3
  Bit Set4 : simulink/Logic and Bit Operations/Bit Set  iBit=7
  Constant7 : Constant  Value=0  OutDataTypeStr=boolean
  Delay2 : Delay  DelayLength=1  InitialCondition=1
  Delay3 : Delay  DelayLength=1  InitialCondition=0
  Switch2 : Switch  Criteria=u2 ~= 0
  Switch3 : Switch  Criteria=u2 ~= 0
  Switch4 : Switch  Criteria=u2 ~= 0
  Dfc_id : Outport  OutDataTypeStr=uint8
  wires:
  Heal/1 -> Switch4/2
  Delay3/1 -> Switch4/3
  Bit Clear1/1 -> Bit Set2/1
  Bit Set2/1 -> Switch4/1
  Err/1 -> Switch3/2
  Switch4/1 -> Switch3/3
  Bit Set/1 -> Bit Set1/1
  Bit Set1/1 -> Switch3/1
  Switch2/1 -> Dfc_id/1, Delay3/1
  Bit Clear2/1 -> Switch2/1
  Switch3/1 -> Switch2/3
  Delay2/1 -> Switch2/2
  Constant7/1 -> Delay2/1
  Bit Set4/1 -> Bit Set/1
  Dfc_id_nv/1 -> Bit Clear1/1, Bit Set4/1, Bit Clear2/1

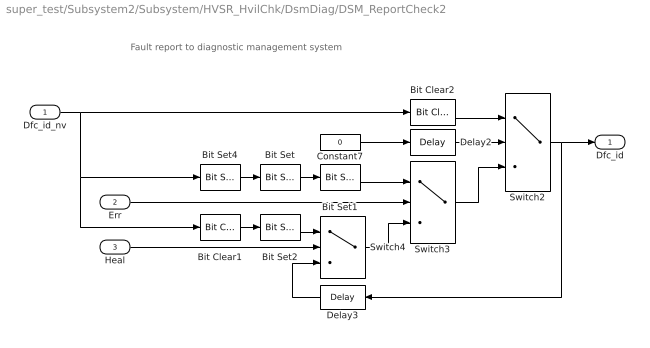
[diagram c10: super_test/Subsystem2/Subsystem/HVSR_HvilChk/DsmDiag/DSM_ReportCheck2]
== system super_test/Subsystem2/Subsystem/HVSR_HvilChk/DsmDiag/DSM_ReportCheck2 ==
  note: Fault report to diagnostic management system
  Dfc_id_nv : Inport  OutDataTypeStr=uint8
  Err : Inport  Port=2
  Heal : Inport  Port=3
  Bit Clear1 : simulink/Logic and Bit Operations/Bit Clear  iBit=4
  Bit Clear2 : simulink/Logic and Bit Operations/Bit Clear  iBit=3
  Bit Set : simulink/Logic and Bit Operations/Bit Set  iBit=4
  Bit Set1 : simulink/Logic and Bit Operations/Bit Set  iBit=3
  Bit Set2 : simulink/Logic and Bit Operations/Bit Set  iBit=3
  Bit Set4 : simulink/Logic and Bit Operations/Bit Set  iBit=7
  Constant7 : Constant  Value=0  OutDataTypeStr=boolean
  Delay2 : Delay  DelayLength=1  InitialCondition=1
  Delay3 : Delay  DelayLength=1  InitialCondition=0
  Switch2 : Switch  Criteria=u2 ~= 0
  Switch3 : Switch  Criteria=u2 ~= 0
  Switch4 : Switch  Criteria=u2 ~= 0
  Dfc_id : Outport  OutDataTypeStr=uint8
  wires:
  Dfc_id_nv/1 -> Bit Clear2/1, Bit Set4/1, Bit Clear1/1
  Bit Set4/1 -> Bit Set/1
  Constant7/1 -> Delay2/1
  Delay2/1 -> Switch2/2
  Switch3/1 -> Switch2/3
  Bit Clear2/1 -> Switch2/1
  Switch2/1 -> Delay3/1, Dfc_id/1
  Bit Set1/1 -> Switch3/1
  Bit Set/1 -> Bit Set1/1
  Switch4/1 -> Switch3/3
  Err/1 -> Switch3/2
  Bit Set2/1 -> Switch4/1
  Bit Clear1/1 -> Bit Set2/1
  Delay3/1 -> Switch4/3
  Heal/1 -> Switch4/2

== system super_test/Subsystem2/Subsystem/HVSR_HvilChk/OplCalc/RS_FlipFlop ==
  S : Inport  OutDataTypeStr=boolean
  R : Inport  Port=2  OutDataTypeStr=boolean
  RS : Stateflow chart  TreatAsAtomicUnit=on
  Q : Outport  OutDataTypeStr=boolean
  !Q : Outport  Port=2  OutDataTypeStr=boolean
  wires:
  R/1 -> RS/2(R)
  S/1 -> RS/1(S)
  RS/2(nQ) -> !Q/1
  RS/1(Q) -> Q/1

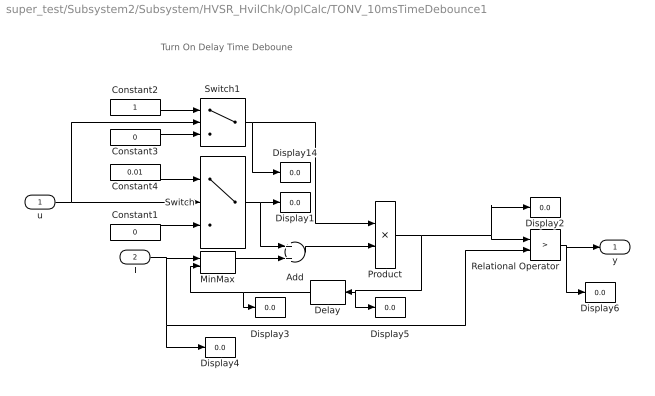
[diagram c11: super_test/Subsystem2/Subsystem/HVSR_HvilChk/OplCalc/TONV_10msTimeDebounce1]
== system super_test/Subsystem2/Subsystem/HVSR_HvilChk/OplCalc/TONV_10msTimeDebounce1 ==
  note: Turn On Delay Time Deboune
  u : Inport
  T : Inport  Port=2
  Add : Sum
  Constant1 : Constant  Value=0  OutDataTypeStr=single
  Constant2 : Constant  OutDataTypeStr=uint8
  Constant3 : Constant  Value=0  OutDataTypeStr=uint8
  Constant4 : Constant  Value=0.01  OutDataTypeStr=single
  Delay : Delay  DelayLength=1  InitialCondition=0
  Display{1..6,14} (7 alike) : Display
  MinMax : MinMax  Inputs=2
  Product : Product  OutMin=[0]  OutMax=[65535]  OutDataTypeStr=single
  Relational Operator : RelationalOperator  Operator=>  OutDataTypeStr=boolean  RndMeth=Simplest
  Switch : Switch  Criteria=u2 ~= 0
  Switch1 : Switch  Criteria=u2 ~= 0
  y : Outport
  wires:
  Switch1/1 -> Display14/1, Product/1
  Constant3/1 -> Switch1/3
  Constant2/1 -> Switch1/1
  u/1 -> Switch1/2, Switch/2
  Constant4/1 -> Switch/1
  Constant1/1 -> Switch/3
  Add/1 -> Product/2
  Product/1 -> Display2/1, Relational Operator/1, Display5/1, Delay/1
  Switch/1 -> Display1/1, Add/1
  Delay/1 -> Display3/1, MinMax/2
  Relational Operator/1 -> Display6/1, y/1
  T/1 -> MinMax/1, Relational Operator/2, Display4/1
  MinMax/1 -> Add/2

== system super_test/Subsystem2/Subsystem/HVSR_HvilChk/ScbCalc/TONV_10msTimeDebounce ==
  note: Turn On Delay Time Deboune
  u : Inport
  T : Inport  Port=2
  Add : Sum
  Constant1 : Constant  Value=0  OutDataTypeStr=single
  Constant2 : Constant  OutDataTypeStr=uint8
  Constant3 : Constant  Value=0  OutDataTypeStr=uint8
  Constant4 : Constant  Value=0.01  OutDataTypeStr=single
  Delay : Delay  DelayLength=1  InitialCondition=0
  MinMax : MinMax  Inputs=2
  Product : Product  OutMin=[0]  OutMax=[65535]  OutDataTypeStr=single
  Relational Operator : RelationalOperator  Operator=>  OutDataTypeStr=boolean  RndMeth=Simplest
  Switch : Switch  Criteria=u2 ~= 0
  Switch1 : Switch  Criteria=u2 ~= 0
  y : Outport
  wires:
  Switch1/1 -> Product/1
  Constant3/1 -> Switch1/3
  Constant2/1 -> Switch1/1
  u/1 -> Switch1/2, Switch/2
  Constant4/1 -> Switch/1
  Constant1/1 -> Switch/3
  Add/1 -> Product/2
  Product/1 -> Relational Operator/1, Delay/1
  Switch/1 -> Add/1
  Delay/1 -> MinMax/2
  Relational Operator/1 -> y/1
  T/1 -> MinMax/1, Relational Operator/2
  MinMax/1 -> Add/2

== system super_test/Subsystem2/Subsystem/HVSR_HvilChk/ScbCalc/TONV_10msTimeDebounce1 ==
  note: Turn On Delay Time Deboune
  u : Inport
  T : Inport  Port=2
  Add : Sum
  Constant1 : Constant  Value=0  OutDataTypeStr=single
  Constant2 : Constant  OutDataTypeStr=uint8
  Constant3 : Constant  Value=0  OutDataTypeStr=uint8
  Constant4 : Constant  Value=0.01  OutDataTypeStr=single
  Delay : Delay  DelayLength=1  InitialCondition=0
  MinMax : MinMax  Inputs=2
  Product : Product  OutMin=[0]  OutMax=[65535]  OutDataTypeStr=single
  Relational Operator : RelationalOperator  Operator=>  OutDataTypeStr=boolean  RndMeth=Simplest
  Switch : Switch  Criteria=u2 ~= 0
  Switch1 : Switch  Criteria=u2 ~= 0
  y : Outport
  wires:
  MinMax/1 -> Add/2
  T/1 -> Relational Operator/2, MinMax/1
  Relational Operator/1 -> y/1
  Delay/1 -> MinMax/2
  Switch/1 -> Add/1
  Product/1 -> Delay/1, Relational Operator/1
  Add/1 -> Product/2
  Constant1/1 -> Switch/3
  Constant4/1 -> Switch/1
  u/1 -> Switch/2, Switch1/2
  Constant2/1 -> Switch1/1
  Constant3/1 -> Switch1/3
  Switch1/1 -> Product/1

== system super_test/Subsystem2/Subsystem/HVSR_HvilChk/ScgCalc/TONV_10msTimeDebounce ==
  note: Turn On Delay Time Deboune
  u : Inport
  T : Inport  Port=2
  Add : Sum
  Constant1 : Constant  Value=0  OutDataTypeStr=single
  Constant2 : Constant  OutDataTypeStr=uint8
  Constant3 : Constant  Value=0  OutDataTypeStr=uint8
  Constant4 : Constant  Value=0.01  OutDataTypeStr=single
  Delay : Delay  DelayLength=1  InitialCondition=0
  MinMax : MinMax  Inputs=2
  Product : Product  OutMin=[0]  OutMax=[65535]  OutDataTypeStr=single
  Relational Operator : RelationalOperator  Operator=>  OutDataTypeStr=boolean  RndMeth=Simplest
  Switch : Switch  Criteria=u2 ~= 0
  Switch1 : Switch  Criteria=u2 ~= 0
  y : Outport
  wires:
  MinMax/1 -> Add/2
  T/1 -> Relational Operator/2, MinMax/1
  Relational Operator/1 -> y/1
  Delay/1 -> MinMax/2
  Switch/1 -> Add/1
  Product/1 -> Delay/1, Relational Operator/1
  Add/1 -> Product/2
  Constant1/1 -> Switch/3
  Constant4/1 -> Switch/1
  u/1 -> Switch/2, Switch1/2
  Constant2/1 -> Switch1/1
  Constant3/1 -> Switch1/3
  Switch1/1 -> Product/1

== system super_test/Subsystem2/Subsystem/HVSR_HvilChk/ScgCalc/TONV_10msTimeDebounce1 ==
  note: Turn On Delay Time Deboune
  u : Inport
  T : Inport  Port=2
  Add : Sum
  Constant1 : Constant  Value=0  OutDataTypeStr=single
  Constant2 : Constant  OutDataTypeStr=uint8
  Constant3 : Constant  Value=0  OutDataTypeStr=uint8
  Constant4 : Constant  Value=0.01  OutDataTypeStr=single
  Delay : Delay  DelayLength=1  InitialCondition=0
  MinMax : MinMax  Inputs=2
  Product : Product  OutMin=[0]  OutMax=[65535]  OutDataTypeStr=single
  Relational Operator : RelationalOperator  Operator=>  OutDataTypeStr=boolean  RndMeth=Simplest
  Switch : Switch  Criteria=u2 ~= 0
  Switch1 : Switch  Criteria=u2 ~= 0
  y : Outport
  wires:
  Switch1/1 -> Product/1
  Constant3/1 -> Switch1/3
  Constant2/1 -> Switch1/1
  u/1 -> Switch1/2, Switch/2
  Constant4/1 -> Switch/1
  Constant1/1 -> Switch/3
  Add/1 -> Product/2
  Product/1 -> Relational Operator/1, Delay/1
  Switch/1 -> Add/1
  Delay/1 -> MinMax/2
  Relational Operator/1 -> y/1
  T/1 -> MinMax/1, Relational Operator/2
  MinMax/1 -> Add/2

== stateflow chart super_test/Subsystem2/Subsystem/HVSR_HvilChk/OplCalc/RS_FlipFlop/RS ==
  state RS_FlipFlop
    (default) -> (junction 3)
    (junction 3) -> (junction 5) : [R]
    (junction 3) -> (junction 12)
    (junction 5) -> (junction 7) : {Q=boolean(0);nQ=boolean(1);}
    (junction 12) -> (junction 14) : [S]
    (junction 14) -> (junction 16) : {Q=boolean(1);nQ=boolean(0);}
    (junction 12) -> (junction 18)
    (junction 16) -> (junction 18)
    (junction 7) -> (junction 18)
    (junction 18) -> (junction 21)
  (default) -> RS_FlipFlop
  (junction 24) -> RS_FlipFlop
  (junction 25) -> (junction 24)
  RS_FlipFlop -> (junction 23)
  (junction 23) -> (junction 25)
  data: S input boolean; R input boolean; Q output boolean; nQ output boolean

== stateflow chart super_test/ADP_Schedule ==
  (default) -> (junction 50)
  (junction 50) -> (junction 13) : { HVSR_HvilChk_step_10ms; BCCR_RlyCtlDiag_step_10ms; }
  events: output FUNCTION_CALL_EVENT; output FUNCTION_CALL_EVENT
